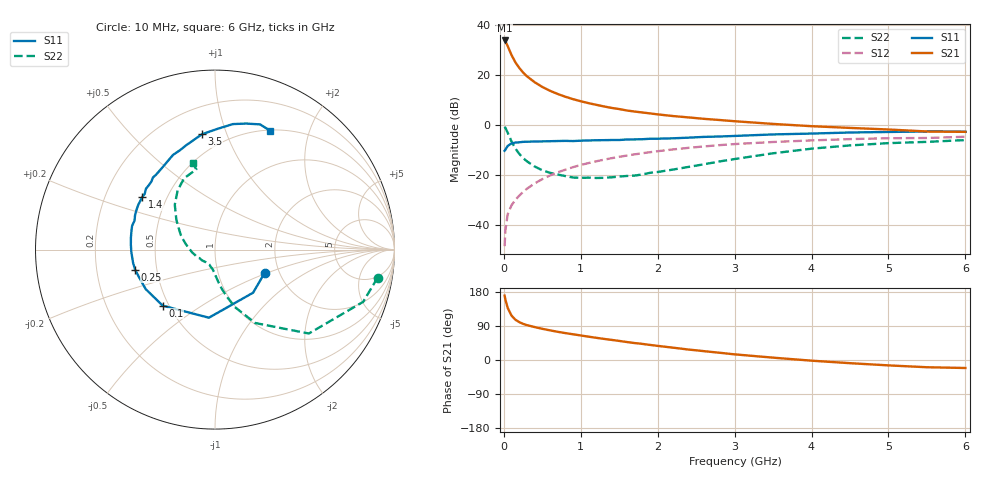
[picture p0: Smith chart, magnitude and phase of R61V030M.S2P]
! SIEMENS Small Signal Semiconductors
! BFR193
! Si NPN RF Bipolar Junction Transistor in SOT23
! VCE = 1 V  IC = 30 mA
! Common Emitter S-Parameters:  May  1996
# GHz  S  MA  R  50
!  f  S11  S21  S12  S22
! GHz  MAG  ANG  MAG  ANG  MAG  ANG  MAG  ANG
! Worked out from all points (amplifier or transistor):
!   36 points, 10 MHz to 6 GHz, reference 50 ohm
!   highest |S21| = 33.7 dB at 10 MHz (marker M1)
!   |S21| within 3 dB of that: start of sweep to 60.71 MHz
!   unconditionally stable (mu >= 1): 399.5 MHz to 2.223 GHz
!   at 250 MHz: K = 0.92, MSG = 23.9 dB, |S12| = -26.8 dB
!   at 1.4 GHz: K = 1.03, MAG = 8.9 dB, |S12| = -13.3 dB
!   at 6 GHz: K = 0.98, MSG = 1.0 dB, |S12| = -4.7 dB
!   S11 on the Smith chart (normalised r, x): 10 MHz: 1.67, -0.48; 100 MHz: 0.46, -0.35; 250 MHz: 0.38, -0.11; 1.4 GHz: 0.36, +0.28; 3.5 GHz: 0.37, +0.82; 6 GHz: 0.51, +1.44
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0.01  0.3053 -25.4  48.58 169.8  0.0038 83.2  0.9192 -9.8
0.02  0.3205 -48.5  46.91 159.8  0.0078 77.2  0.8755 -19.4
0.05  0.381 -95.1  37.58 137.5  0.0165 66.7  0.7015 -41.8
0.1  0.4271 -133.0  24.83 117.1  0.0249 63.1  0.4663 -61.3
0.15  0.4446 -150.4  17.8 106.3  0.032 63.0  0.3382 -71.0
0.2  0.4498 -159.7  13.78 100.0  0.0387 66.0  0.2653 -76.3
0.25  0.4592 -166.0  11.15 95.4  0.0459 66.8  0.219 -80.4
0.3  0.4625 -171.2  9.371 92.0  0.0532 69.0  0.1879 -83.4
0.4  0.4663 -178.3  7.136 86.9  0.068 69.8  0.1483 -88.3
0.5  0.4696 176.6  5.732 82.3  0.0827 70.2  0.1242 -92.8
0.6  0.4732 171.9  4.81 78.2  0.0979 69.9  0.1108 -96.8
0.7  0.4774 167.0  4.151 74.4  0.1131 69.4  0.1024 -101.2
0.9  0.4765 160.2  3.27 67.9  0.1437 67.3  0.0892 -110.5
1.1  0.4898 153.4  2.726 61.6  0.1731 64.9  0.0886 -119.5
1.4  0.4999 144.1  2.188 53.1  0.2167 60.4  0.09 -134.2
1.7  0.5146 135.7  1.851 44.7  0.2585 55.9  0.0975 -150.5
2.2  0.5411 123.5  1.504 32.5  0.3245 47.9  0.1286 -173.2
3  0.6029 105.5  1.186 14.9  0.415 34.6  0.2085 156.6
3.5  0.6465 96.5  1.048 6.2  0.4565 26.5  0.2714 142.5
4.5  0.7063 81.9  0.872 -8.4  0.5214 12.4  0.3903 122.2
5.5  0.7414 70.2  0.74 -19.1  0.5489 -1.1  0.4591 103.1
6  0.7302 65.1  0.728 -21.1  0.5811 -5.1  0.4986 104.5
